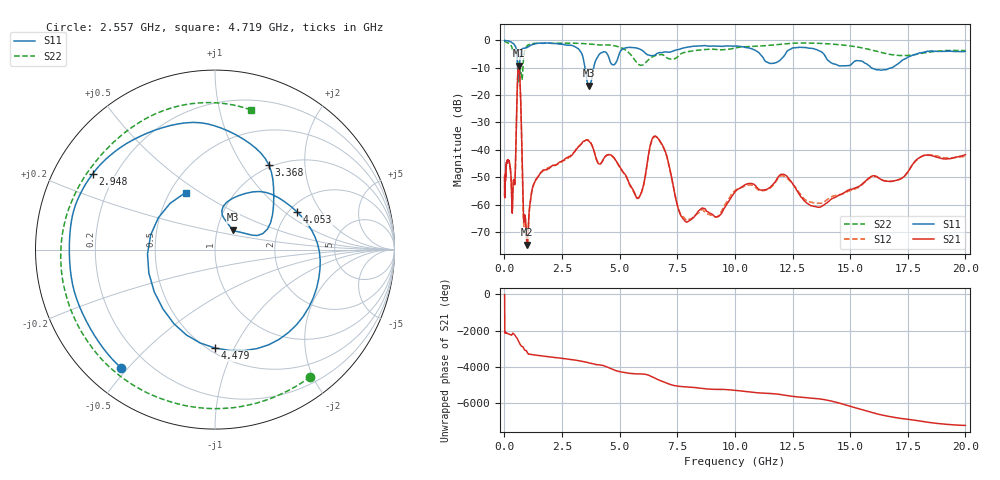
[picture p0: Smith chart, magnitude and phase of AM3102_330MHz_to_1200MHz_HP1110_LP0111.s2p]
! Date/Time: Tue, Sep 11, 2018 5:23 PM
! Network Analyzer: Agilent Technologies E8362B Rev: A.07.50.63
! Sweep from 0.010 to 20.000 GHz, 1601 Points, Sweep Type: LOG
! Power Supply: 4.949 V, 0.001 A
# Hz S DB R 50
!freq MagS11 AngS11 MagS21 AngS21 MagS12 AngS12 MagS22 AngS22
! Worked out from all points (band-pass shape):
!   1601 points, 10 MHz to 20 GHz, reference 50 ohm
!   highest |S21| = -9.29 dB at 617.7 MHz (marker M1); lowest = -74.7 dB at 984 MHz (marker M2)
!   |S21| within 3 dB of the highest: 580.7 MHz to 661.4 MHz (80.72 MHz wide, 13 % of centre)
!   lowest |S11| = -16.6 dB at 3.668 GHz (marker M3), VSWR 1.35, Z = 59.2 + j13.4 ohm
!   |S11| at or under -10 dB: 570.4 MHz to 647.3 MHz (76.92 MHz wide, 12.6 % of centre); 3.497 GHz to 3.875 GHz (377.8 MHz wide, 10.2 % of centre); 15.92 GHz to 16.8 GHz (886.1 MHz wide, 5.42 % of centre)
!   |S22| runs from -15.7 to -0.1 dB; largest |S21 - S12| = 0.0054
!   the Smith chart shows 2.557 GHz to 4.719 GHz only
!   S11 on the Smith chart (normalised r, x): 2.557 GHz: 0.11, -0.48; 2.948 GHz: 0.12, +0.28; 3.368 GHz: 0.97, +1.32; 4.053 GHz: 2.20, +1.24; 4.479 GHz: 0.54, -0.84; 4.719 GHz: 0.60, +0.44
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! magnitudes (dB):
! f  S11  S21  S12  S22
! 10 MHz  0.0  -49.7  -49.7  -0.1
! 35.55 MHz  -0.1  -51.2  -51.5  -0.4
! 126.4 MHz  -0.2  -44.3  -44.2  -0.9
! 256.5 MHz  -0.5  -46.8  -46.9  -1.5
! 337.9 MHz  -1.0  -62.7  -62.8  -2.8
! 447.2 MHz  -1.8  -52.8  -52.4  -4.2
! 617.7 MHz  -13.4  -9.3  -9.4  -14.6
! 702.3 MHz  -4.9  -20.5  -20.5  -10.5
! 833.3 MHz  -2.9  -65.0  -66.6  -6.6
! 984 MHz  -2.6  -74.7  -75.0  -2.0
! 1.59 GHz  -1.1  -48.2  -48.2  -1.0
! 2.557 GHz  -1.5  -43.9  -44.0  -1.1
! 2.948 GHz  -1.9  -41.8  -41.5  -1.1
! 3.368 GHz  -5.1  -37.5  -37.6  -1.2
! 3.668 GHz  -16.6  -36.8  -36.6  -1.3
! 4.053 GHz  -6.0  -44.8  -44.5  -1.7
! 4.479 GHz  -5.2  -41.9  -41.8  -1.7
! 4.719 GHz  -8.9  -42.6  -42.7  -1.9
! 5.652 GHz  -2.7  -55.8  -56.2  -7.1
! 6.58 GHz  -5.1  -35.1  -35.3  -5.5
! 7.958 GHz  -2.5  -66.2  -65.7  -4.1
! 20 GHz  -4.1  -41.8  -42.4  -3.7
